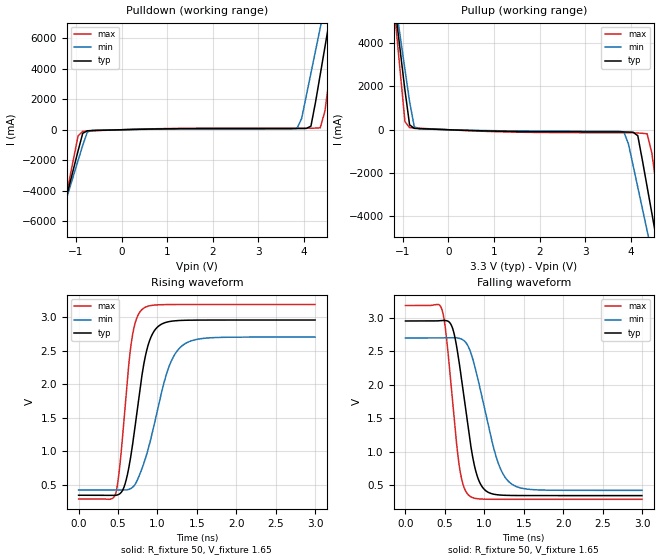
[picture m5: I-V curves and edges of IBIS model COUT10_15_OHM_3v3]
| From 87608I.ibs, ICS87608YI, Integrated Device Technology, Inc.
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[Model] COUT10_15_OHM_3v3
Model_type   Output
Polarity   Non-Inverting
Vmeas = 1.65
Rref = 50
Cref = 0
Vref = 1.65
|   typ   min   max
C_comp   2pF   1.5pF   2.5pF
|   typ   min   max
[Voltage range]  3.3V   3.135V   3.465V
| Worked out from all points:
|   slope of the pulldown table from 0 to 0.495 V, typ, clamps not added: 13.8 ohm
|   slope of the pullup table from 0 to 0.495 V, typ, clamps not added: 13.7 ohm
|   rising waveform, R_fixture 50, V_fixture 1.65: 20-80 % time 196ps typ, 298ps min, 137ps max; typ from 0.341 V to 2.96 V
|   falling waveform, R_fixture 50, V_fixture 1.65: 20-80 % time 193ps typ, 277ps min, 144ps max; typ from 2.96 V to 0.341 V
[pulldown]
|Voltage   I (typ)   I (min)   I (max)
-3.3V     -29.16A    -25.15A    -35.86A
-1.463V   -7.429A    -7.049A    -8.123A
-1.361V   -6.221A    -6.044A    -6.58A
-952.6mV  -1.39A     -2.025A    -405.5mA
-850.5mV  -234.5mA   -1.022A    -103.8mA
-646.4mV  -52.93mA   -43.23mA   -68.97mA
3.844V    79.54mA    85.8mA     101.9mA
4.151V    235.2mA    3.716A     103.7mA
4.355V    3.628A     6.703A     124.5mA
4.559V    7.219A     9.692A     3.517A
4.763V    10.81A     12.68A     8.113A
6.6V      43.31A     39.72A     49.65A
[pullup]
|Voltage   I (typ)   I (min)   I (max)
-3.3V     43.25A     37.27A     53.27A
-1.157V   5.426A     5.787A     4.935A
-952.6mV  1.827A     2.793A     380.1mA
-850.5mV  222.5mA    1.296A     95.37mA
-748.5mV  65.22mA    142.1mA    80.97mA
-646.4mV  53.41mA    42.85mA    69.61mA
3.844V    -102.2mA   -100.2mA   -139.3mA
4.151V    -277.4mA   -2.661A    -152.1mA
4.355V    -2.633A    -4.664A    -188.6mA
4.559V    -5.043A    -6.67A     -2.6A
4.763V    -7.453A    -8.676A    -5.681A
6.6V      -29.16A    -26.75A    -33.4A
[Ramp]
|   typ   min   max
dV/dt_r   2.093/0.305n   1.826/0.463n   2.325/0.212n
dV/dt_f   2.098/0.289n   1.829/0.416n   2.333/0.215n
[Rising Waveform]
R_fixture = 50
V_fixture = 1.65
V_fixture_max = 1.73
V_fixture_min = 1.57
C_fixture = 0.0p
| Time   typ   min   max
0s        340.7mV    419.1mV    284.7mV
465ps     339.1mV    419.2mV    348.2mV
514.6ps   356.7mV    418.6mV    695.2mV
576.6ps   464.6mV    417.6mV    1.477V
672.7ps   1.005V     448.4mV    2.651V
812.2ps   2.197V     766.3mV    3.121V
973.4ps   2.816V     1.47V      3.179V
1.144ns   2.931V     2.253V     3.186V
1.324ns   2.951V     2.581V     3.187V
2.998ns   2.955V     2.701V     3.187V
[Falling Waveform]
R_fixture = 50
V_fixture = 1.65
V_fixture_max = 1.73
V_fixture_min = 1.57
C_fixture = 0.0p
| Time   typ   min   max
0s        2.955V     2.701V     3.187V
461.9ps   2.963V     2.701V     3.127V
511.5ps   2.961V     2.701V     2.792V
589ps     2.873V     2.705V     1.86V
682ps     2.322V     2.696V     785mV
809.1ps   1.236V     2.539V     338.5mV
970.3ps   475.6mV    1.818V     288.3mV
1.163ns   353.1mV    873.6mV    285mV
1.327ns   342.9mV    531mV      284.7mV
2.998ns   340.7mV    419.1mV    284.7mV
